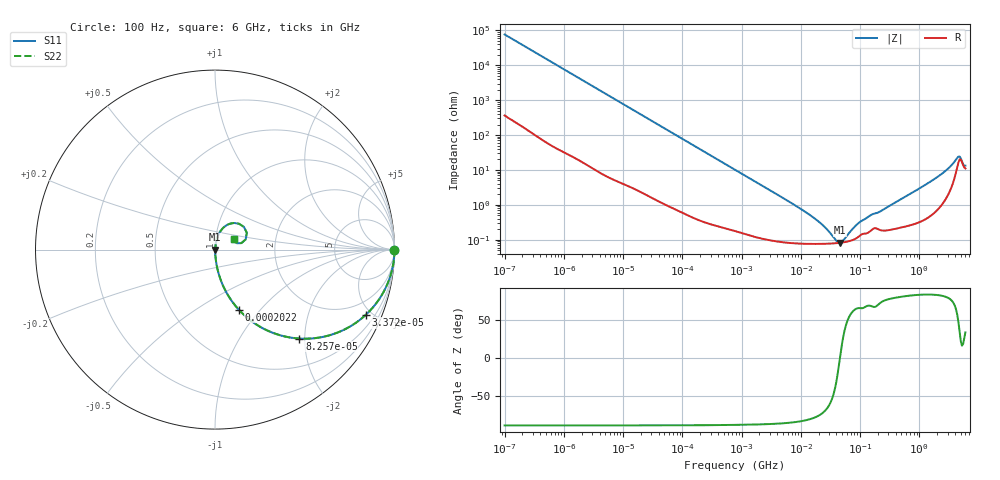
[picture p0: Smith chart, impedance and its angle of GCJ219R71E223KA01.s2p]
!Murata Part Number: GCJ219R71E223KA01
!These Parameters are Measured in Series Mode Connection
!Data Generated on Mar 13, 2026
!  o--ll--o
!Port1  Port2
!  o------o
!Operation Temp=25[degC], DC Bias Voltage=0[V]
!Freq. Start=100[Hz] Stop=6[GHz] 401[Steps]
# Hz S RI R 50
!Freq.(Hz) S11(Real) S11(Imag) S21(Real) S21(Imag) S12(Real) S12(Imag) S22(Real) S22(Imag)
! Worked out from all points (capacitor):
!   401 points, 100 Hz to 6 GHz, reference 50 ohm
!   read as one part in series: C = 20.9 nF near 109 Hz
!   lowest |Z| = 81.8 mohm at 45.56 MHz (marker M1)
!   series resonance near 45.81 MHz, so ESL is about 580 pH
!   S11 on the Smith chart (normalised r, x): 100 Hz: open; 33.72 kHz: 1.03, -4.59; 82.57 kHz: 1.01, -1.88; 202.2 kHz: 1.01, -0.77; 6 GHz: 1.22, +0.15
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100  1 -0.00131  8e-06 0.00131  8e-06 0.00131  1 -0.00131
2008  0.9992 -0.0261  0.0008 0.0261  0.0008 0.0261  0.9992 -0.0261
9626  0.984 -0.1228  0.016 0.1228  0.016 0.1228  0.984 -0.1228
19704  0.9377 -0.2387  0.0623 0.2387  0.0623 0.2387  0.9377 -0.2387
33721  0.8391 -0.3643  0.1609 0.3643  0.1609 0.3643  0.8391 -0.3643
40335  0.7854 -0.4073  0.2146 0.4073  0.2146 0.4073  0.7854 -0.4073
82567  0.4701 -0.4954  0.5299 0.4954  0.5299 0.4954  0.4701 -0.4954
202169  0.1318 -0.3338  0.8682 0.3338  0.8682 0.3338  0.1318 -0.3338
345986  0.0508 -0.2139  0.9492 0.2139  0.9492 0.2139  0.0508 -0.2139
774597  0.0119 -0.1001  0.9881 0.1001  0.9881 0.1001  0.0119 -0.1001
1.555665e7  0.000781 -0.00454  0.9992 0.00454  0.9992 0.00454  0.000781 -0.00454
2.545746e7  0.000771 -0.00217  0.9992 0.00217  0.9992 0.00217  0.000771 -0.00217
3.983537e7  0.000799 -0.000489  0.9992 0.000489  0.9992 0.000489  0.000799 -0.000489
4.556224e7  0.000818 -1.84e-05  0.9992 1.84e-05  0.9992 1.84e-05  0.000818 -1.84e-05
5.211241e7  0.000843 0.000452  0.9992 -0.000452  0.9992 -0.000452  0.000843 0.000452
9.753859e7  0.00128 0.00288  0.9987 -0.00288  0.9987 -0.00288  0.00128 0.00288
3.124326e8  0.00198 0.00909  0.998 -0.00909  0.998 -0.00909  0.00198 0.00909
1.95892e9  0.0103 0.0593  0.9897 -0.0593  0.9897 -0.0593  0.0103 0.0593
3.352442e9  0.0401 0.1155  0.9599 -0.1155  0.9599 -0.1155  0.0401 0.1155
4.385646e9  0.1331 0.1444  0.8669 -0.1444  0.8669 -0.1444  0.1331 0.1444
4.796499e9  0.1775 0.0935  0.8225 -0.0935  0.8225 -0.0935  0.1775 0.0935
6e9  0.1032 0.0598  0.8968 -0.0598  0.8968 -0.0598  0.1032 0.0598
